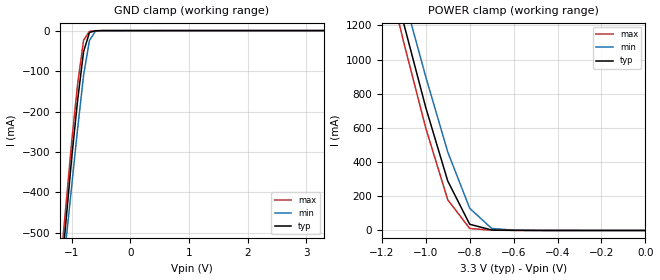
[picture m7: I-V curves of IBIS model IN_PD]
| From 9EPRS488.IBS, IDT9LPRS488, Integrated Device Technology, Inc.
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|   Model IN_PD
[Model]   IN_PD
Model_type   Input
Polarity   Inverting
Vinl =   0.80V
Vinh =   2.00V
C_comp   3.40pF   2.85pF   3.95pF
[Temperature Range]   27.00   70.00   0.000
[Voltage Range]   3.30V   3.00V   3.70V
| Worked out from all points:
|   GND clamp passes 1 mA (typ) near -0.61 V on its own axis
|   POWER clamp passes 1 mA (typ) near -0.61 V on its own axis
[GND_clamp]
| voltage   I(typ)   I(min)   I(max)
-3.3V     -4.16A     -4.01A     -4.26A
-1.2V     -630mA     -670mA     -590mA
-1.1V     -470mA     -520mA     -430mA
-1V       -310mA     -380mA     -270mA
-900mV    -170mA     -240mA     -130mA
-800mV    -52.21mA   -110mA     -23.66mA
-700mV    -4.72mA    -24.36mA   -1.88mA
-600mV    -450uA     -1.92mA    -240uA
-500mV    -55.23uA   -160uA     -38.19uA
3.3V      36.64uA    48.37uA    55.23uA
[POWER_clamp]
| voltage   I(typ)   I(min)   I(max)
-3.3V     13.35A     12.84A     13.68A
-1.2V     1.72A      1.85A      1.63A
-1.1V     1.21A      1.37A      1.1A
-1V       720mA      900mA      600mA
-900mV    290mA      460mA      180mA
-800mV    36.38mA    130mA      11.72mA
-700mV    2.87mA     12.1mA     1.58mA
-600mV    800uA      1.77mA     490uA
0V        36.64nA    24.18nA    55.37nA
